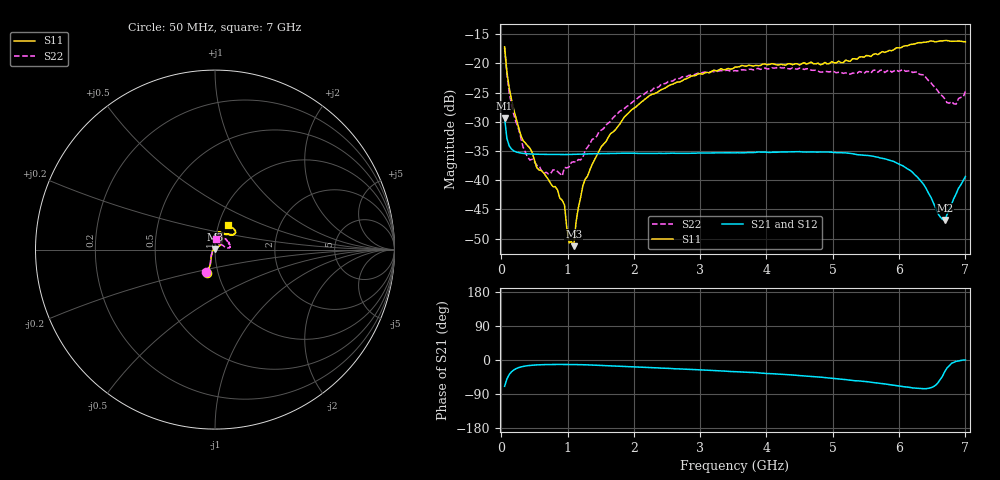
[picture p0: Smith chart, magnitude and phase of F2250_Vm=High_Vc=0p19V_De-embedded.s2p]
! Integrated Device Technology
! Corporate Headquarters
! 6024 Silver Creek Valley Road
! San Jose, CA 95138  USA
! Phone:  1-408-284-8200
! Toll Free:  1-800-223-1366
! Webpage:  http://www.idt.com/
! Timing and RF Division
! 515 Groton Road, Suite 102
! Westford, MA 01886-6024
! Device:  F2250
! Description: Voltage Variable RF Attenuator
! Frequency:  50.0 -  6000.00 MHz
! Package:  3x3 mm Thin QFN Plastic Package: 16 pin
! Ports:  2 RF, 3 DC
!  Pin  1  = GND
!  Pin  2  = NC
!  Pin  3  = RF1  = Port 1
!  Pin  4  = NC
!  Pin  5  = GND
!  Pin  6  = GND
!  Pin  7  = GND
!  Pin  8  = GND
!  Pin  9  = NC
!  Pin 10  = RF2  = Port 2
!  Pin 11  = NC
!  Pin 12  = GND
!  Pin 13  = GND
!  Pin 14  = VCNTRL
!  Pin 15  = VDD
!  Pin 16  = VMODE
! Vcntrl:  0.190 Volts
! Vmode:  +3.300 Volts
! Vdd:  +3.30  Volts
! Current:  1.244 mA
! Data:  The device was measured on a the F2250 evaluation board which has
!  individual transmission lines to the RF pins.  Data was collected
!  using a calibrated network analyzer.  The evaluation board was
!  de-embedded using a TRL calibration technique.
!  The reference plane is the edge of the package pin.
! Misc:  SN 10
!  Action Tracker AT0258
! Date Measured:  2014-11-26
! Date:  2015-10-15  MJV
! Note:
!  Integrated Device Technology supplies this data as a sample of measured
!  data at the package pin for this product.  Your particular data for this
!  product may vary.
!  Data was taken at 25 degrees C.
!  Integrated Device Technology reserves the right to change this data at anytime.
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# GHz S dB R 50
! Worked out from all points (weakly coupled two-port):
!   201 points, 50 MHz to 7 GHz, reference 50 ohm
!   highest |S21| = -29.38 dB at 50 MHz (marker M1); lowest = -46.8 dB at 6.687 GHz (marker M2)
!   lowest |S11| = -51.3 dB at 1.093 GHz (marker M3), VSWR 1.01, Z = 50 + j0.273 ohm
!   |S11| at or under -10 dB: start of sweep to end of sweep
!   |S22| runs from -39.2 to -17.4 dB; largest |S21 - S12| = 6.3e-05
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0.05  -17.18 -108.5  -29.38 -69.5  -29.38 -69.5  -17.37 -110.6
0.08475  -21.48 -107.4  -32.86 -50.1  -32.86 -50.1  -21.87 -109.0
0.15425  -26.23 -116.5  -34.68 -31.0  -34.68 -31.0  -27.11 -120.6
0.29325  -32.27 -127.5  -35.35 -18.4  -35.35 -18.5  -32.67 -133.6
0.3975  -34.11 -142.1  -35.48 -15.0  -35.48 -15.0  -36.07 -158.5
0.5365  -37.88 -154.5  -35.55 -12.9  -35.55 -12.9  -37.47 -180.0
0.64075  -38.78 -162.4  -35.57 -12.2  -35.58 -12.2  -38.87 160.6
0.91875  -43.42 155.9  -35.60 -11.8  -35.60 -11.8  -39.24 127.8
0.9535  -44.24 171.0  -35.60 -11.8  -35.60 -11.8  -37.81 124.2
1.023  -50.69 140.3  -35.59 -11.9  -35.59 -11.9  -37.71 108.2
1.0925  -51.27 89.4  -35.57 -12.0  -35.57 -12.0  -36.84 98.7
1.12725  -47.18 61.6  -35.56 -12.1  -35.57 -12.2  -36.91 91.7
1.2315  -40.87 40.9  -35.53 -12.5  -35.52 -12.5  -36.06 77.3
1.6485  -32.02 41.3  -35.44 -15.2  -35.44 -15.2  -29.93 60.0
2.37825  -24.76 46.7  -35.40 -21.0  -35.40 -21.1  -24.02 53.9
3.525  -20.65 71.8  -35.32 -30.6  -35.32 -30.7  -21.26 72.9
4.7065  -20.07 72.0  -35.15 -43.9  -35.15 -43.9  -21.21 70.4
5.85325  -17.79 40.5  -36.58 -64.8  -36.57 -65.0  -21.13 23.4
6.27025  -16.53 39.4  -39.39 -74.5  -39.40 -74.5  -21.46 8.6
6.68725  -16.11 47.8  -46.81 -31.0  -46.78 -30.8  -26.03 28.4
6.861  -16.22 54.5  -42.31 -3.7  -42.27 -3.7  -26.97 57.4
7  -16.32 62.4  -39.36 -0.0  -39.32 -0.3  -24.82 83.6
